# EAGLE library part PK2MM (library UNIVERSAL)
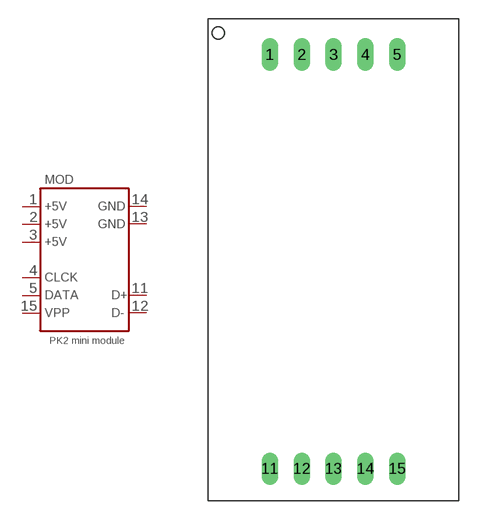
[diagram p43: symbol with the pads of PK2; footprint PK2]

Designator prefix MOD

## PK2MM  [PK2]
1  1  pwr
2  2  pwr
3  3  pwr
4  4
5  5
11  11
12  12
13  13  pwr
14  14  pwr
15  15  out

## Footprint PK2 (pad centres in mm)
drill 0.8 long: 1 0,33.02; 2 2.54,33.02; 3 5.08,33.02; 4 7.62,33.02; 5 10.16,33.02; 11 0,0; 12 2.54,0; 13 5.08,0; 14 7.62,0; 15 10.16,0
